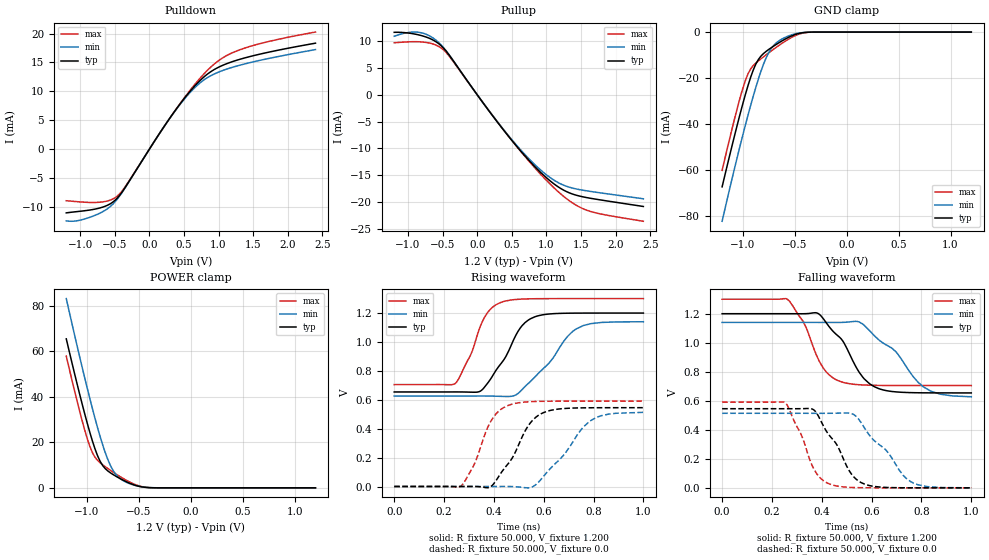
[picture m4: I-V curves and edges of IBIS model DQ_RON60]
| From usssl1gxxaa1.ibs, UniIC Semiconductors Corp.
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|   Model DQ_RON60
[Model] DQ_RON60
Model_type I/O
Vinl =  0.500V
Vinh =  0.700V
Vmeas =  0.600V
Rref =  50.000
Vref =  0.600V
C_comp   1.373pF   1.353pF   1.403pF
[Model Spec]
Vinh   0.700V   0.670V   0.750V
Vinl   0.500V   0.470V   0.550V
Vmeas   0.600V   0.570V   0.650V
Vref   0.600V   0.570V   0.650V
Rref   50.000   NA   NA
[Temperature Range]   25.000   0.125k   -40.000
[Voltage Range]   1.200V   1.140V   1.300V
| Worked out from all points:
|   slope of the pulldown table from 0 to 0.18 V, typ, clamps not added: 53.9 ohm
|   slope of the pullup table from 0 to 0.18 V, typ, clamps not added: 56.5 ohm
|   GND clamp passes 1 mA (typ) near -0.49 V on its own axis
|   POWER clamp passes 1 mA (typ) near -0.53 V on its own axis
|   rising waveform, R_fixture 50.000, V_fixture 1.200: 20-80 % time 110ps typ, 147ps min, 85.5ps max; typ from 0.654 V to 1.2 V
|   rising waveform, R_fixture 50.000, V_fixture 0.0: 20-80 % time 110ps typ, 143ps min, 85ps max; typ from 0 V to 0.545 V
|   falling waveform, R_fixture 50.000, V_fixture 1.200: 20-80 % time 125ps typ, 168ps min, 96.1ps max; typ from 1.2 V to 0.654 V
|   falling waveform, R_fixture 50.000, V_fixture 0.0: 20-80 % time 110ps typ, 147ps min, 86.1ps max; typ from 0.545 V to 0 V
[Pulldown]
|Voltage   I(typ)   I(min)   I(max)
-1.2V     -11mA      -12.39mA   -8.906mA
-1.015V   -10.74mA   -12.3mA    -9.094mA
-756mV    -10.28mA   -11.28mA   -9.188mA
-571mV    -9.478mA   -9.976mA   -8.824mA
-460mV    -8.406mA   -8.587mA   -8.076mA
-349mV    -6.601mA   -6.657mA   -6.475mA
354mV     6.371mA    6.322mA    6.372mA
613mV     10.37mA    10.13mA    10.56mA
798mV     12.6mA     12.06mA    13.14mA
1.02V     14.3mA     13.44mA    15.49mA
1.316V    15.58mA    14.56mA    17.24mA
2.4V      18.34mA    17.23mA    20.27mA
[Pullup]
|Voltage   I(typ)   I(min)   I(max)
-1.2V     11.68mA    10.95mA    9.732mA
-1.004V   11.56mA    11.63mA    9.897mA
-819mV    11.12mA    11.63mA    9.898mA
-634mV    10.21mA    10.58mA    9.478mA
-486mV    8.716mA    8.811mA    8.386mA
106mV     -1.891mA   -1.877mA   -1.865mA
513mV     -8.73mA    -8.588mA   -8.729mA
846mV     -13.6mA    -13.22mA   -13.85mA
1.142V    -16.96mA   -16.21mA   -17.78mA
1.364V    -18.48mA   -17.39mA   -20.1mA
1.586V    -19.21mA   -17.95mA   -21.58mA
2.4V      -20.87mA   -19.43mA   -23.63mA
[GND_clamp]
|Voltage   I(typ)   I(min)   I(max)
-1.2V     -67.26mA   -82.22mA   -60.1mA
-1.05V    -39.62mA   -53.62mA   -32.4mA
-1V       -31.05mA   -44.64mA   -24.37mA
-950mV    -23.16mA   -36.01mA   -18.1mA
-925mV    -19.62mA   -31.85mA   -16.02mA
-875mV    -13.89mA   -23.97mA   -13.48mA
-800mV    -9.288mA   -13.81mA   -10.72mA
-750mV    -7.535mA   -8.829mA   -8.993mA
-675mV    -5.274mA   -4.578mA   -6.506mA
-525mV    -1.587mA   -1.138mA   -2.208mA
-375mV    -90.13uA   -87.27uA   -132.9uA
1.2V      0A         0A         0A
[POWER_clamp]
|Voltage   I(typ)   I(min)   I(max)
-1.2V     65.51mA    83.21mA    57.91mA
-1.05V    37.38mA    53.57mA    29.99mA
-1V       28.74mA    44.18mA    21.95mA
-950mV    20.85mA    35.16mA    15.65mA
-925mV    17.34mA    30.84mA    13.56mA
-875mV    11.74mA    22.7mA     11.06mA
-800mV    7.436mA    12.47mA    8.502mA
-750mV    5.864mA    7.69mA     6.933mA
-675mV    3.901mA    3.837mA    4.735mA
-525mV    971.5uA    903.1uA    1.25mA
-400mV    85.95uA    125.9uA    91.19uA
1.2V      0A         0A         0A
[Ramp]
| variable   typ   min   max
dV/dt_r   0.327/0.110n   0.308/0.143n   0.354/85.039p
dV/dt_f   0.328/0.125n   0.308/0.168n   0.357/96.296p
R_load = 50.000
[Rising Waveform]
R_fixture= 50.000
V_fixture= 1.200
V_fixture_min= 1.140
V_fixture_max= 1.300
|time   V(typ)   V(min)   V(max)
0s        654.1mV    625.8mV    705.1mV
244ps     654.2mV    625.8mV    711.7mV
310ps     652.5mV    625.9mV    923.6mV
346ps     660mV      626mV      1.11V
378ps     721.7mV    625.8mV    1.211V
431ps     855.6mV    623.5mV    1.275V
505ps     1.094V     655.9mV    1.296V
563ps     1.173V     754.3mV    1.299V
729ps     1.2V       1.089V     1.3V
1ns       1.2V       1.14V      1.3V
[Rising Waveform]
R_fixture= 50.000
V_fixture= 0.0
V_fixture_min= 0.0
V_fixture_max= 0.0
|time   V(typ)   V(min)   V(max)
0s        47.48nV    824nV      27.71nV
267ps     31.45uV    454.4nV    1.056mV
319ps     280.2uV    -14.78uV   144.9mV
381ps     -6.83mV    49.8uV     429.5mV
421ps     73.34mV    282uV      523.8mV
462ps     167.3mV    94.79uV    563.9mV
540ps     425.1mV    -9.135mV   586.1mV
599ps     511.1mV    69.49mV    589.6mV
785ps     544.7mV    452.5mV    590.7mV
1ns       545.3mV    513mV      590.8mV
[Falling Waveform]
R_fixture= 50.000
V_fixture= 1.200
V_fixture_min= 1.140
V_fixture_max= 1.300
|time   V(typ)   V(min)   V(max)
0s        1.2V       1.14V      1.3V
262ps     1.2V       1.14V      1.3V
324ps     1.2V       1.14V      1.15V
380ps     1.205V     1.14V      909.2mV
447ps     1.076V     1.14V      755.4mV
550ps     796.6mV    1.143V     710.4mV
635ps     680.1mV    1.011V     705.9mV
700ps     660.8mV    933.5mV    705.3mV
807ps     654.8mV    696.8mV    705.1mV
1ns       654.1mV    627.5mV    705.1mV
[Falling Waveform]
R_fixture= 50.000
V_fixture= 0.0
V_fixture_min= 0.0
V_fixture_max= 0.0
|time   V(typ)   V(min)   V(max)
0s        545.3mV    513.7mV    590.8mV
251ps     545.2mV    513.7mV    588.7mV
315ps     545.5mV    513.7mV    376.3mV
363ps     542.2mV    513.6mV    147.5mV
397ps     458.7mV    513.5mV    63.06mV
435ps     351.6mV    513.9mV    23.93mV
528ps     76.11mV    505.3mV    2.193mV
573ps     24.78mV    408.4mV    693.3uV
755ps     239uV      44.53mV    6.404uV
1ns       488.1nV    111.7uV    27.61nV
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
